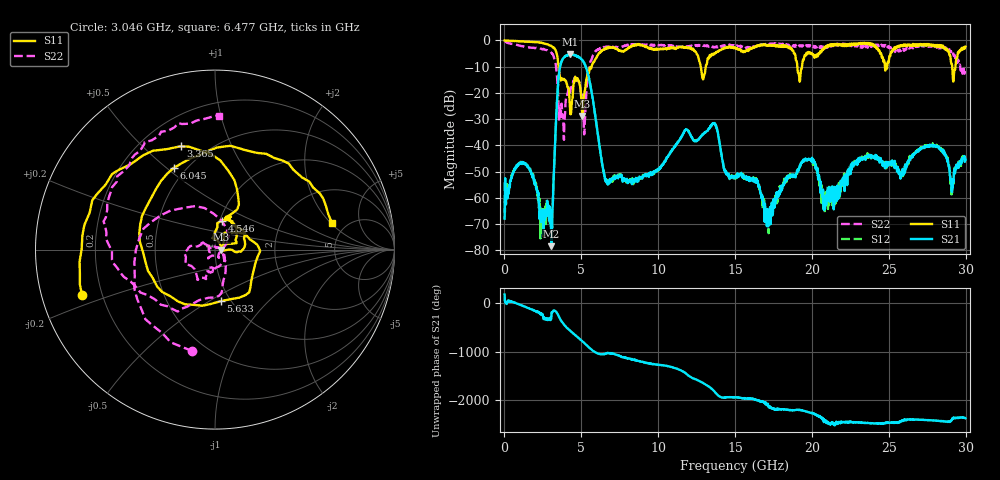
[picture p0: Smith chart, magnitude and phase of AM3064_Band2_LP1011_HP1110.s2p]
# Hz S DB R 50.0
!freq dBS11 angS11 dBS21 angS21 dBS12 angS12 dBS22 angS22
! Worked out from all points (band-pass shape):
!   1600 points, 10 MHz to 29.98 GHz, reference 50 ohm
!   highest |S21| = -5.25 dB at 4.246 GHz (marker M1); lowest = -78.4 dB at 3.046 GHz (marker M2)
!   |S21| within 3 dB of the highest: 3.696 GHz to 5.144 GHz (1.448 GHz wide, 32.8 % of centre)
!   lowest |S11| = -28.8 dB at 5.071 GHz (marker M3), VSWR 1.07, Z = 53.7 - j0.112 ohm
!   |S11| at or under -10 dB: 3.515 GHz to 5.666 GHz (2.151 GHz wide, 46.9 % of centre); 12.77 GHz to 13.09 GHz (327.7 MHz wide, 2.53 % of centre); 19.05 GHz to 19.35 GHz (303.2 MHz wide, 1.58 % of centre)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
!   |S22| runs from -37.9 to -0.3 dB; largest |S21 - S12| = 0.012
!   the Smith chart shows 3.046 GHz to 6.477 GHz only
!   S11 on the Smith chart (normalised r, x): 3.046 GHz: 0.13, -0.16; 3.365 GHz: 0.36, +0.66; 4.546 GHz: 1.03, +0.34; 5.633 GHz: 0.90, -0.57; 6.045 GHz: 0.43, +0.53; 6.477 GHz: 3.86, +2.07
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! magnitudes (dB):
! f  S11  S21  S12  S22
! 10 MHz  0.0  -67.9  -54.1  -0.3
! 1.191 GHz  -0.4  -46.6  -47.1  -2.3
! 3.046 GHz  -2.1  -78.4  -72.0  -4.7
! 3.365 GHz  -4.3  -29.5  -29.5  -10.7
! 3.777 GHz  -14.9  -7.3  -7.3  -29.2
! 4.246 GHz  -24.7  -5.2  -5.3  -19.7
! 4.546 GHz  -15.6  -5.6  -5.5  -14.8
! 5.015 GHz  -24.5  -7.2  -7.2  -21.5
! 5.071 GHz  -28.8  -7.6  -7.6  -21.2
! 5.633 GHz  -10.8  -18.5  -18.4  -7.7
! 6.045 GHz  -5.8  -34.6  -34.4  -3.6
! 6.477 GHz  -3.5  -50.6  -50.9  -2.5
! 10 GHz  -3.4  -49.4  -48.9  -1.9
! 13.6 GHz  -5.1  -31.8  -31.5  -2.5
! 15 GHz  -2.8  -51.7  -52.4  -1.9
! 16.34 GHz  -2.5  -52.9  -53.2  -2.5
! 17.16 GHz  -2.0  -70.9  -66.0  -1.4
! 19.2 GHz  -15.8  -47.7  -48.6  -2.2
! 19.99 GHz  -4.9  -46.2  -45.8  -1.9
! 20.89 GHz  -2.3  -61.1  -60.5  -2.8
! 25 GHz  -8.0  -46.4  -46.7  -2.3
! 29.98 GHz  -2.4  -45.5  -44.4  -10.3
